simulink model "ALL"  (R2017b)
settings: Solver=VariableStepAuto  StartTime=0.0  StopTime=30  RelTol=1e-3
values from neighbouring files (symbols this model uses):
  Ce = 0.33    [init.m]
  Cm = 0.33    [init.m]
  DL = 10    [init.m]
  g_az_b_x = p10    [run_simu.m]
  g_az_b_y = p11    [run_simu.m]
  g_pi_az_x = p12    [run_simu.m]
  g_pi_az_z = p13    [run_simu.m]
  JLa = 0.04    [init.m]
  JLp = 0.02    [init.m]
  Jma = 0.02    [init.m]
  Jmp = 0.01    [init.m]
  Kg = 15/pi    (= 4.77464829276)    [init.m]
  KL = 100000    [init.m]
  Kp = 20    [init.m]
  lg = 0.7    [init.m]
  Lm = 0.01    [init.m]
  r_az_b_x = p6    [run_simu.m]
  r_az_b_y = p7    [run_simu.m]
  r_pi_az_x = p8    [run_simu.m]
  r_pi_az_z = p9    [run_simu.m]
  Rc = 0.4    [init.m]
  Rm = 8.6    [init.m]
  uav_dis_fre = p1    [run_simu.m]
  v_az_b_x = p2    [run_simu.m]
  v_az_b_y = p3    [run_simu.m]
  v_pi_az_x = p4    [run_simu.m]
  v_pi_az_z = p5    [run_simu.m]
  wg = 200*pi    (= 628.318530718)    [init.m]

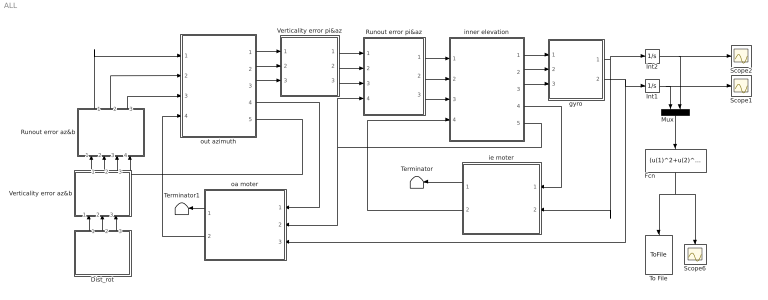
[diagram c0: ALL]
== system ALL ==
  Dist_rot : Subsystem
  Fcn : Fcn  Expr=(u(1)^2+u(2)^2)^0.5
  Int1 : Integrator
  Int2 : Integrator
  Mux : Mux  Inputs=2
  Runout error az&b : Subsystem
  Runout error pi&az : Subsystem
  Scope1 : Scope
  Scope2 : Scope
  Scope6 : Scope
  Terminator : Terminator
  Terminator1 : Terminator
  To File : ToFile  Filename=result.mat  MatrixName=accuracy  SaveFormat=Timeseries
  Verticality error az&b : Subsystem
  Verticality error pi&az : Subsystem
  gyro : Subsystem
  ie moter : Subsystem
  inner elevation : Subsystem
  oa moter : Subsystem
  out azimuth : Subsystem
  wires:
  out azimuth/4(Tacho Out) -> oa moter/1(In aztacho)
  inner elevation/4(Tacho Out) -> ie moter/1(In pitacho)
  oa moter/2(Out az abvel) -> out azimuth/4(V ab)
  ie moter/2(Out pi abvel) -> inner elevation/4(V ab)
  inner elevation/5(Angle Out) -> oa moter/2(In piangle), Runout error pi&az/4(Wibz1)
  inner elevation/1(X  OUT) -> gyro/1(Wipx)
  inner elevation/2(Y  OUT (GYRO)) -> gyro/2(Wipy)
  inner elevation/3(Z  OUT) -> gyro/3(Wipz)
  gyro/2(X  OUT Az) -> Int1/1, oa moter/3(In azgyro)
  gyro/1(Y  OUT Az) -> Int2/1, ie moter/2(In pigyro)
  Mux/1 -> Fcn/1
  Fcn/1 -> Scope6/1, To File/1
  out azimuth/5(Angle Out) -> Runout error az&b/4(Wibz1)
  Runout error az&b/2(Wiby') -> out azimuth/2(In Y)
  Runout error az&b/1(Wibx'1) -> out azimuth/1(In X)
  Runout error az&b/3(Wibz') -> out azimuth/3(In Z)
  out azimuth/2(Y  OUT) -> Verticality error pi&az/2(Wiay)
  out azimuth/1(X  OUT) -> Verticality error pi&az/1(Wiax)
  out azimuth/3(Z  OUT (GYRO)) -> Verticality error pi&az/3(Wiaz)
  Verticality error pi&az/1(Wiax'1) -> Runout error pi&az/1(Wiax)
  Verticality error pi&az/2(Wiay') -> Runout error pi&az/2(Wiay)
  Verticality error pi&az/3(Wiaz') -> Runout error pi&az/3(Wiaz)
  Runout error pi&az/2(Wiay') -> inner elevation/2(In Y)
  Runout error pi&az/1(Wiax'1) -> inner elevation/1(In X)
  Runout error pi&az/3(Wiaz') -> inner elevation/3(In Z)
  Verticality error az&b/2(Wiby') -> Runout error az&b/2(Wiby)
  Verticality error az&b/1(Wibx'1) -> Runout error az&b/1(Wibx)
  Verticality error az&b/3(Wibz') -> Runout error az&b/3(Wibz)
  Dist_rot/2(Out2) -> Verticality error az&b/2(Wiby)
  Dist_rot/1(Out1) -> Verticality error az&b/1(Wibx)
  Dist_rot/3(Out3) -> Verticality error az&b/3(Wibz)
  Int2/1 -> Mux/2, Scope2/1
  Int1/1 -> Mux/1, Scope1/1
  oa moter/1(Out az torque) -> Terminator1/1
  ie moter/1(Out pi torque) -> Terminator/1

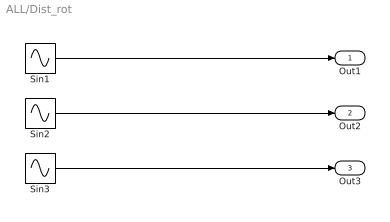
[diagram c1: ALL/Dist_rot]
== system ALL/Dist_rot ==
  Sin1 : Sin  Amplitude=pi/180*1.5  Frequency=pi*2*uav_dis_fre  SampleTime=0
  Sin2 : Sin  Amplitude=pi/180*1.5  Frequency=pi*2*uav_dis_fre  SampleTime=0
  Sin3 : Sin  Amplitude=pi/180*1.5  Frequency=2*pi*uav_dis_fre  SampleTime=0
  Out1 : Outport
  Out2 : Outport  Port=2
  Out3 : Outport  Port=3
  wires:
  Sin2/1 -> Out2/1
  Sin3/1 -> Out3/1
  Sin1/1 -> Out1/1

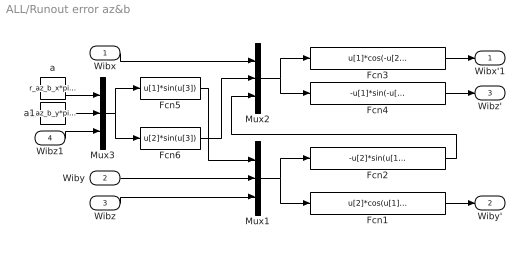
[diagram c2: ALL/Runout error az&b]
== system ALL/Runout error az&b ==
  Wibx : Inport
  Wiby : Inport  Port=2
  Wibz : Inport  Port=3
  Wibz1 : Inport  Port=4
  Fcn1 : Fcn  Expr=u[2]*cos(u[1])+u[3]*sin(u[1])
  Fcn2 : Fcn  Expr=-u[2]*sin(u[1])+u[3]*cos(u[1])
  Fcn3 : Fcn  Expr=u[1]*cos(-u[2])+u[3]*sin(-u[2])
  Fcn4 : Fcn  Expr=-u[1]*sin(-u[2])+u[3]*cos(-u[2])
  Fcn5 : Fcn  Expr=u[1]*sin(u[3])
  Fcn6 : Fcn  Expr=u[2]*sin(u[3])
  Mux1 : Mux  Inputs=3
  Mux2 : Mux  Inputs=3
  Mux3 : Mux  Inputs=3
  a : Constant  Value=r_az_b_x*pi/180
  a1 : Constant  Value=r_az_b_y*pi/180
  Wibx'1 : Outport
  Wiby' : Outport  Port=2
  Wibz' : Outport  Port=3
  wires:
  Mux3/1 -> Fcn6/1, Fcn5/1
  Fcn4/1 -> Wibz'/1
  Fcn1/1 -> Wiby'/1
  Fcn3/1 -> Wibx'1/1
  Fcn2/1 -> Mux2/3
  Fcn5/1 -> Mux1/1
  Mux2/1 -> Fcn3/1, Fcn4/1
  Wiby/1 -> Mux1/2
  Wibx/1 -> Mux2/1
  Fcn6/1 -> Mux2/2
  a1/1 -> Mux3/2
  Mux1/1 -> Fcn1/1, Fcn2/1
  Wibz/1 -> Mux1/3
  Wibz1/1 -> Mux3/3
  a/1 -> Mux3/1

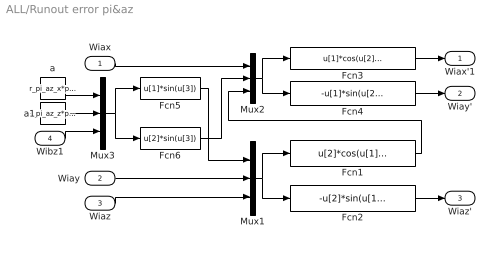
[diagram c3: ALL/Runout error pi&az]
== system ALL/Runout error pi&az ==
  Wiax : Inport
  Wiay : Inport  Port=2
  Wiaz : Inport  Port=3
  Wibz1 : Inport  Port=4
  Fcn1 : Fcn  Expr=u[2]*cos(u[1])+u[3]*sin(u[1])
  Fcn2 : Fcn  Expr=-u[2]*sin(u[1])+u[3]*cos(u[1])
  Fcn3 : Fcn  Expr=u[1]*cos(u[2])+u[3]*sin(u[2])
  Fcn4 : Fcn  Expr=-u[1]*sin(u[2])+u[3]*cos(u[2])
  Fcn5 : Fcn  Expr=u[1]*sin(u[3])
  Fcn6 : Fcn  Expr=u[2]*sin(u[3])
  Mux1 : Mux  Inputs=3
  Mux2 : Mux  Inputs=3
  Mux3 : Mux  Inputs=3
  a : Constant  Value=r_pi_az_x*pi/180
  a1 : Constant  Value=r_pi_az_z*pi/180
  Wiax'1 : Outport
  Wiay' : Outport  Port=2
  Wiaz' : Outport  Port=3
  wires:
  Mux1/1 -> Fcn2/1, Fcn1/1
  Wiaz/1 -> Mux1/3
  Fcn2/1 -> Wiaz'/1
  Fcn1/1 -> Mux2/3
  Fcn5/1 -> Mux1/1
  Wibz1/1 -> Mux3/3
  Fcn3/1 -> Wiax'1/1
  Mux2/1 -> Fcn4/1, Fcn3/1
  Mux3/1 -> Fcn6/1, Fcn5/1
  a/1 -> Mux3/1
  Fcn6/1 -> Mux2/2
  Wiay/1 -> Mux1/2
  a1/1 -> Mux3/2
  Fcn4/1 -> Wiay'/1
  Wiax/1 -> Mux2/1

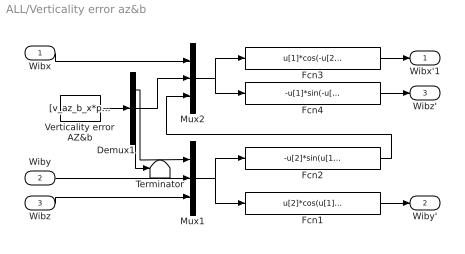
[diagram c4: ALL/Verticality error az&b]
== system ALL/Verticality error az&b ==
  Wibx : Inport
  Wiby : Inport  Port=2
  Wibz : Inport  Port=3
  Demux1 : Demux  Outputs=3
  Fcn1 : Fcn  Expr=u[2]*cos(u[1])+u[3]*sin(u[1])
  Fcn2 : Fcn  Expr=-u[2]*sin(u[1])+u[3]*cos(u[1])
  Fcn3 : Fcn  Expr=u[1]*cos(-u[2])+u[3]*sin(-u[2])
  Fcn4 : Fcn  Expr=-u[1]*sin(-u[2])+u[3]*cos(-u[2])
  Mux1 : Mux  Inputs=3
  Mux2 : Mux  Inputs=3
  Terminator : Terminator
  Verticality error AZ&b : Constant  Value=[v_az_b_x*pi/180 v_az_b_y*pi/180 0*pi/180]'
  Wibx'1 : Outport
  Wiby' : Outport  Port=2
  Wibz' : Outport  Port=3
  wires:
  Verticality error AZ&b/1 -> Demux1/1
  Fcn3/1 -> Wibx'1/1
  Wibx/1 -> Mux2/1
  Demux1/2 -> Mux2/2
  Demux1/1 -> Mux1/1
  Mux1/1 -> Fcn1/1, Fcn2/1
  Fcn1/1 -> Wiby'/1
  Wibz/1 -> Mux1/3
  Fcn2/1 -> Mux2/3
  Wiby/1 -> Mux1/2
  Fcn4/1 -> Wibz'/1
  Mux2/1 -> Fcn3/1, Fcn4/1
  Demux1/3 -> Terminator/1

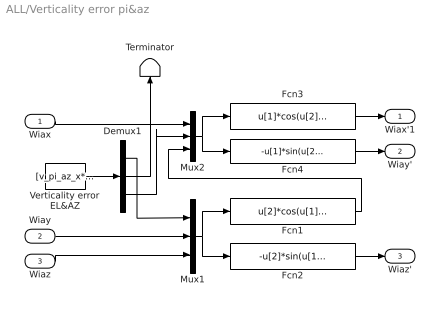
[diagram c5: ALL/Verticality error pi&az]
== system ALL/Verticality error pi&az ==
  Wiax : Inport
  Wiay : Inport  Port=2
  Wiaz : Inport  Port=3
  Demux1 : Demux  Outputs=3
  Fcn1 : Fcn  Expr=u[2]*cos(u[1])+u[3]*sin(u[1])
  Fcn2 : Fcn  Expr=-u[2]*sin(u[1])+u[3]*cos(u[1])
  Fcn3 : Fcn  Expr=u[1]*cos(u[2])+u[3]*sin(u[2])
  Fcn4 : Fcn  Expr=-u[1]*sin(u[2])+u[3]*cos(u[2])
  Mux1 : Mux  Inputs=3
  Mux2 : Mux  Inputs=3
  Terminator : Terminator
  Verticality error EL&AZ : Constant  Value=[v_pi_az_x*pi/180 0*pi/180 v_pi_az_z*pi/180]'  VectorParams1D=off
  Wiax'1 : Outport
  Wiay' : Outport  Port=2
  Wiaz' : Outport  Port=3
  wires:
  Wiax/1 -> Mux2/1
  Fcn4/1 -> Wiay'/1
  Demux1/1 -> Mux1/1
  Fcn3/1 -> Wiax'1/1
  Mux2/1 -> Fcn4/1, Fcn3/1
  Fcn1/1 -> Mux2/3
  Fcn2/1 -> Wiaz'/1
  Wiay/1 -> Mux1/2
  Mux1/1 -> Fcn2/1, Fcn1/1
  Demux1/3 -> Mux2/2
  Wiaz/1 -> Mux1/3
  Verticality error EL&AZ/1 -> Demux1/1
  Demux1/2 -> Terminator/1

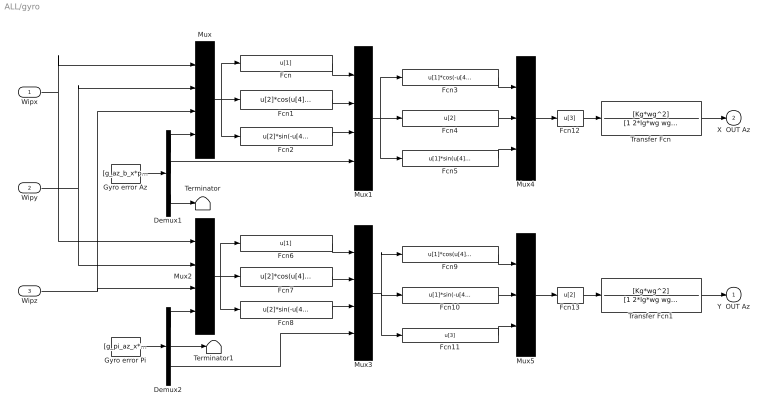
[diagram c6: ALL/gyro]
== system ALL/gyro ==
  Wipx : Inport
  Wipy : Inport  Port=2
  Wipz : Inport  Port=3
  Demux1 : Demux  Outputs=3
  Demux2 : Demux  Outputs=3
  Fcn : Fcn  Expr=u[1]
  Fcn1 : Fcn  Expr=u[2]*cos(u[4])+u[3]*sin(u[4])
  Fcn10 : Fcn  Expr=u[1]*sin(-u[4])+u[2]*cos(u[4])
  Fcn11 : Fcn  Expr=u[3]
  Fcn12 : Fcn  Expr=u[3]
  Fcn13 : Fcn  Expr=u[2]
  Fcn2 : Fcn  Expr=u[2]*sin(-u[4])+u[3]*cos(u[4])
  Fcn3 : Fcn  Expr=u[1]*cos(-u[4])+u[3]*sin(-u[4])
  Fcn4 : Fcn  Expr=u[2]
  Fcn5 : Fcn  Expr=u[1]*sin(u[4])+u[3]*cos(u[4])
  Fcn6 : Fcn  Expr=u[1]
  Fcn7 : Fcn  Expr=u[2]*cos(u[4])+u[3]*sin(u[4])
  Fcn8 : Fcn  Expr=u[2]*sin(-u[4])+u[3]*cos(u[4])
  Fcn9 : Fcn  Expr=u[1]*cos(u[4])+u[2]*sin(u[4])
  Gyro error Az : Constant  Value=[g_az_b_x*pi/180 g_az_b_y*pi/180 0*pi/180]'
  Gyro error Pi : Constant  Value=[g_pi_az_x*pi/180 0*pi/180 g_pi_az_z*pi/180]'
  Mux{,1..3} (4 alike) : Mux
  Mux4 : Mux  Inputs=3
  Mux5 : Mux  Inputs=3
  Terminator : Terminator
  Terminator1 : Terminator
  Transfer Fcn : TransferFcn  Numerator=[Kg*wg^2]  Denominator=[1 2*lg*wg wg^2]
  Transfer Fcn1 : TransferFcn  Numerator=[Kg*wg^2]  Denominator=[1 2*lg*wg wg^2]
  Y  OUT Az : Outport
  X  OUT Az : Outport  Port=2
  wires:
  Mux1/1 -> Fcn3/1, Fcn4/1, Fcn5/1
  Fcn1/1 -> Mux1/2
  Fcn12/1 -> Transfer Fcn/1
  Mux5/1 -> Fcn13/1
  Gyro error Pi/1 -> Demux2/1
  Fcn13/1 -> Transfer Fcn1/1
  Fcn3/1 -> Mux4/1
  Fcn4/1 -> Mux4/2
  Fcn10/1 -> Mux5/2
  Fcn9/1 -> Mux5/1
  Fcn8/1 -> Mux3/3
  Mux/1 -> Fcn/1, Fcn1/1, Fcn2/1
  Fcn7/1 -> Mux3/2
  Mux4/1 -> Fcn12/1
  Demux1/1 -> Mux/4
  Mux2/1 -> Fcn8/1, Fcn7/1, Fcn6/1
  Demux2/3 -> Mux3/4
  Mux3/1 -> Fcn9/1, Fcn10/1, Fcn11/1
  Fcn/1 -> Mux1/1
  Fcn5/1 -> Mux4/3
  Fcn6/1 -> Mux3/1
  Demux1/2 -> Mux1/4
  Demux2/1 -> Mux2/4
  Transfer Fcn/1 -> X  OUT Az/1
  Fcn11/1 -> Mux5/3
  Gyro error Az/1 -> Demux1/1
  Fcn2/1 -> Mux1/3
  Transfer Fcn1/1 -> Y  OUT Az/1
  Wipx/1 -> Mux2/1, Mux/1
  Wipy/1 -> Mux2/2, Mux/2
  Wipz/1 -> Mux2/3, Mux/3
  Demux1/3 -> Terminator/1
  Demux2/2 -> Terminator1/1

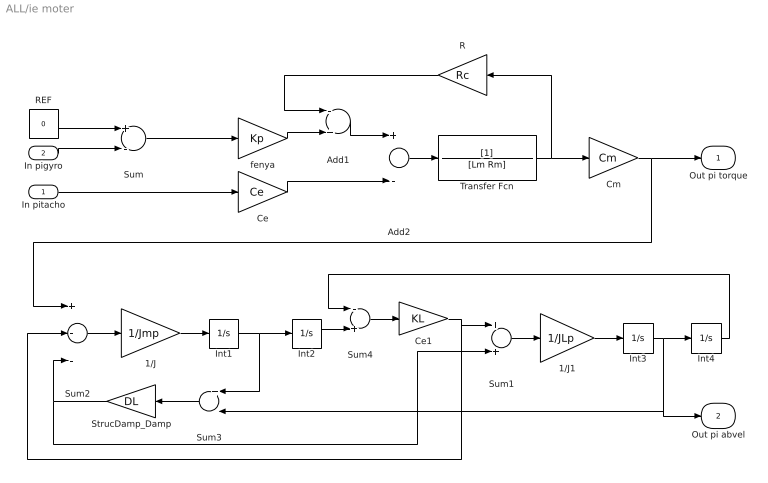
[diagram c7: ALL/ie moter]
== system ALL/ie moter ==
  In pitacho : Inport
  In pigyro : Inport  Port=2
  1/J : Gain  Gain=1/Jmp
  1/J1 : Gain  Gain=1/JLp
  Add1 : Sum  Inputs=-+
  Add2 : Sum  Inputs=+-
  Ce : Gain  Gain=Ce
  Ce1 : Gain  Gain=KL
  Cm : Gain  Gain=Cm
  Int{1..4} (4 alike) : Integrator
  R : Gain  Gain=Rc
  REF : Constant  Value=0
  StrucDamp_Damp : Gain  Gain=DL
  Sum : Sum  Inputs=+-
  Sum1 : Sum
  Sum2 : Sum  Inputs=+--
  Sum3 : Sum  Inputs=+-
  Sum4 : Sum  Inputs=-+
  Transfer Fcn : TransferFcn  Denominator=[Lm Rm]
  fenya : Gain  Gain=Kp
  Out pi torque : Outport
  Out pi abvel : Outport  Port=2
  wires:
  Ce1/1 -> Sum1/1, Sum2/2
  Sum1/1 -> 1/J1/1
  1/J1/1 -> Int3/1
  StrucDamp_Damp/1 -> Sum1/2, Sum2/3
  Int3/1 -> Int4/1, Out pi abvel/1, Sum3/2
  Int4/1 -> Sum4/1
  Int2/1 -> Sum4/2
  Ce/1 -> Add2/2
  Sum3/1 -> StrucDamp_Damp/1
  Cm/1 -> Out pi torque/1, Sum2/1
  1/J/1 -> Int1/1
  Sum2/1 -> 1/J/1
  fenya/1 -> Add1/2
  Int1/1 -> Sum3/1, Int2/1
  Add1/1 -> Add2/1
  R/1 -> Add1/1
  Add2/1 -> Transfer Fcn/1
  Transfer Fcn/1 -> R/1, Cm/1
  REF/1 -> Sum/1
  Sum/1 -> fenya/1
  In pigyro/1 -> Sum/2
  Sum4/1 -> Ce1/1
  In pitacho/1 -> Ce/1

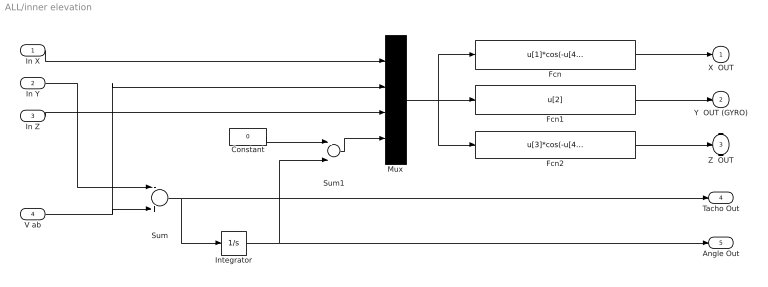
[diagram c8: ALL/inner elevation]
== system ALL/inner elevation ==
  In X : Inport
  In Y : Inport  Port=2
  In Z : Inport  Port=3
  V ab : Inport  Port=4
  Constant : Constant  Value=0
  Fcn : Fcn  Expr=u[1]*cos(-u[4])+u[3]*sin(-u[4])
  Fcn1 : Fcn  Expr=u[2]
  Fcn2 : Fcn  Expr=u[3]*cos(-u[4])-u[1]*sin(-u[4])
  Integrator : Integrator
  Mux : Mux
  Sum : Sum  Inputs=-+
  Sum1 : Sum
  X  OUT : Outport
  Y  OUT (GYRO) : Outport  Port=2
  Z  OUT : Outport  Port=3
  Tacho Out : Outport  Port=4
  Angle Out : Outport  Port=5
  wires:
  In Y/1 -> Sum/1
  Sum/1 -> Integrator/1, Tacho Out/1
  Constant/1 -> Sum1/1
  Sum1/1 -> Mux/4
  Fcn2/1 -> Z  OUT/1
  Fcn/1 -> X  OUT/1
  Mux/1 -> Fcn/1, Fcn2/1, Fcn1/1
  Fcn1/1 -> Y  OUT (GYRO)/1
  Integrator/1 -> Sum1/2, Angle Out/1
  V ab/1 -> Sum/2, Mux/2
  In Z/1 -> Mux/3
  In X/1 -> Mux/1

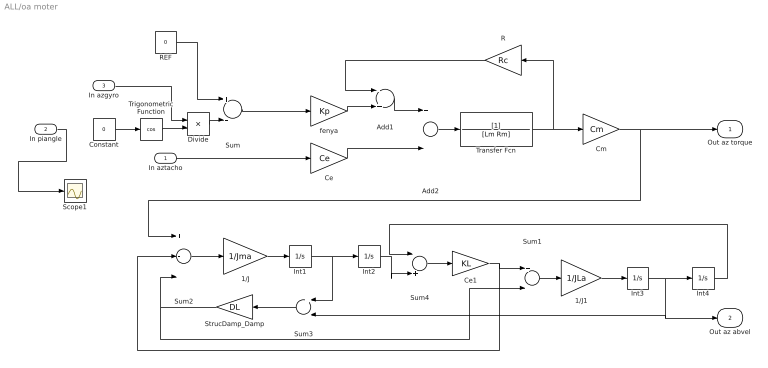
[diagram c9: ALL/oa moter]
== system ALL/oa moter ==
  In aztacho : Inport
  In piangle : Inport  Port=2
  In azgyro : Inport  Port=3
  1/J : Gain  Gain=1/Jma
  1/J1 : Gain  Gain=1/JLa
  Add1 : Sum  Inputs=-+
  Add2 : Sum  Inputs=+-
  Ce : Gain  Gain=Ce
  Ce1 : Gain  Gain=KL
  Cm : Gain  Gain=Cm
  Constant : Constant  Value=0
  Divide : Product  Inputs=*/
  Int{1..4} (4 alike) : Integrator
  R : Gain  Gain=Rc
  REF : Constant  Value=0
  Scope1 : Scope
  StrucDamp_Damp : Gain  Gain=DL
  Sum : Sum  Inputs=+-
  Sum1 : Sum
  Sum2 : Sum  Inputs=+--
  Sum3 : Sum  Inputs=+-
  Sum4 : Sum  Inputs=-+
  Transfer Fcn : TransferFcn  Denominator=[Lm Rm]
  Trigonometric Function : Trigonometry  Operator=cos
  fenya : Gain  Gain=Kp
  Out az torque : Outport
  Out az abvel : Outport  Port=2
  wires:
  Ce1/1 -> Sum2/2, Sum1/1
  Sum1/1 -> 1/J1/1
  1/J1/1 -> Int3/1
  StrucDamp_Damp/1 -> Sum1/2, Sum2/3
  Int3/1 -> Out az abvel/1, Sum3/2, Int4/1
  Int4/1 -> Sum4/1
  Int2/1 -> Sum4/2
  Ce/1 -> Add2/2
  Sum3/1 -> StrucDamp_Damp/1
  Cm/1 -> Sum2/1, Out az torque/1
  1/J/1 -> Int1/1
  Sum2/1 -> 1/J/1
  fenya/1 -> Add1/2
  Int1/1 -> Sum3/1, Int2/1
  Add1/1 -> Add2/1
  R/1 -> Add1/1
  Add2/1 -> Transfer Fcn/1
  Transfer Fcn/1 -> R/1, Cm/1
  REF/1 -> Sum/1
  Sum/1 -> fenya/1
  Sum4/1 -> Ce1/1
  In aztacho/1 -> Ce/1
  In azgyro/1 -> Divide/1
  Trigonometric Function/1 -> Divide/2
  Divide/1 -> Sum/2
  Constant/1 -> Trigonometric Function/1
  In piangle/1 -> Scope1/1

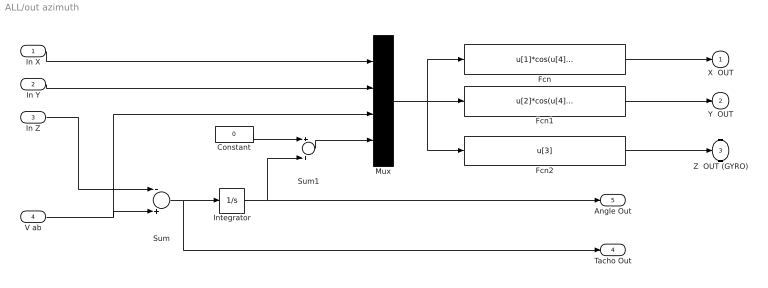
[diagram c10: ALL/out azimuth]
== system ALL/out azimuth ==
  In X : Inport
  In Y : Inport  Port=2
  In Z : Inport  Port=3
  V ab : Inport  Port=4
  Constant : Constant  Value=0
  Fcn : Fcn  Expr=u[1]*cos(u[4])+u[2]*sin(u[4])
  Fcn1 : Fcn  Expr=u[2]*cos(u[4])-u[1]*sin(u[4])
  Fcn2 : Fcn  Expr=u[3]
  Integrator : Integrator
  Mux : Mux
  Sum : Sum  Inputs=-+
  Sum1 : Sum
  X  OUT : Outport
  Y  OUT : Outport  Port=2
  Z  OUT (GYRO) : Outport  Port=3
  Tacho Out : Outport  Port=4
  Angle Out : Outport  Port=5
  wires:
  Sum/1 -> Tacho Out/1, Integrator/1
  Constant/1 -> Sum1/1
  Sum1/1 -> Mux/4
  Integrator/1 -> Angle Out/1, Sum1/2
  V ab/1 -> Mux/3, Sum/2
  In X/1 -> Mux/1
  Fcn1/1 -> Y  OUT/1
  Fcn2/1 -> Z  OUT (GYRO)/1
  Mux/1 -> Fcn/1, Fcn1/1, Fcn2/1
  Fcn/1 -> X  OUT/1
  In Z/1 -> Sum/1
  In Y/1 -> Mux/2
